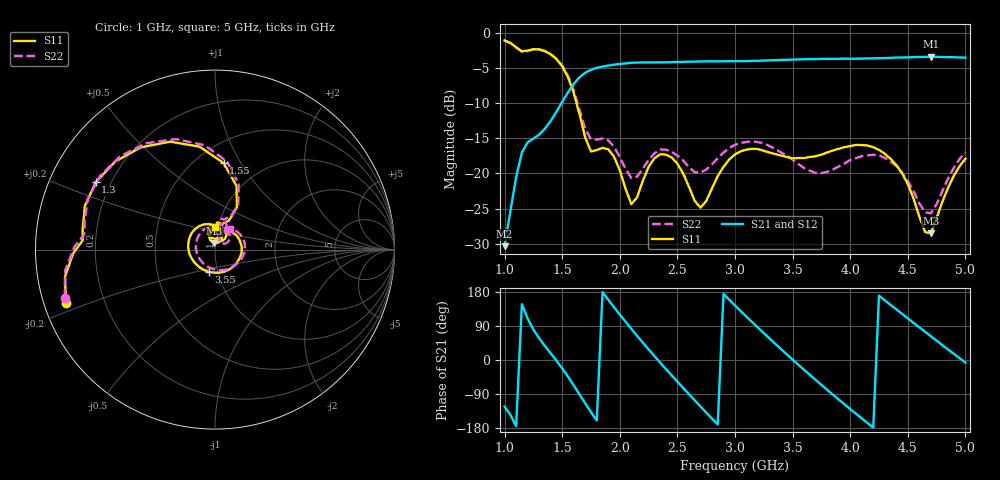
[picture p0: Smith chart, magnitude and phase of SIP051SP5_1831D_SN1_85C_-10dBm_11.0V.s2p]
# GHz  S  dB  R  50
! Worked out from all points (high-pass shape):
!   81 points, 1 GHz to 5 GHz, reference 50 ohm
!   highest |S21| = -3.41 dB at 4.7 GHz (marker M1); lowest = -30.3 dB at 1 GHz (marker M2)
!   |S21| within 3 dB of the highest: 1.645 GHz to end of sweep
!   lowest |S11| = -28.5 dB at 4.7 GHz (marker M3), VSWR 1.08, Z = 49.4 + j3.69 ohm
!   |S11| at or under -10 dB: 1.624 GHz to end of sweep
!   |S22| runs from -25.7 to -1.1 dB; largest |S21 - S12| = 0.0021
!   S11 on the Smith chart (normalised r, x): 1 GHz: 0.06, -0.17; 1.3 GHz: 0.14, +0.26; 1.55 GHz: 0.67, +0.85; 3.55 GHz: 0.91, -0.23; 5 GHz: 0.96, +0.25
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1  -1.08 -160.3  -30.34 -123.1  -30.30 -123.0  -1.10 -162.0
1.15  -2.62 176.1  -17.02 147.1  -16.99 147.3  -2.69 173.4
1.3  -2.35 150.6  -14.48 57.4  -14.47 57.3  -2.37 147.4
1.55  -6.30 84.3  -8.47 -43.9  -8.47 -43.9  -6.12 82.1
1.7  -14.91 64.2  -5.66 -114.5  -5.66 -114.6  -13.66 64.6
1.85  -16.35 85.1  -4.80 179.2  -4.79 179.3  -15.04 77.1
2.05  -22.18 68.4  -4.35 100.9  -4.34 101.0  -19.34 63.9
2.2  -21.04 112.2  -4.21 45.7  -4.21 45.7  -19.32 89.0
2.35  -17.28 90.2  -4.20 -6.6  -4.18 -6.5  -16.60 76.3
2.5  -18.61 58.6  -4.16 -57.1  -4.13 -57.1  -17.47 55.2
2.65  -23.89 50.8  -4.09 -106.3  -4.07 -106.3  -19.81 52.6
2.85  -20.38 75.8  -4.06 -170.1  -4.04 -170.1  -17.82 57.6
3  -17.28 45.1  -4.04 144.0  -4.03 144.0  -15.92 38.3
3.25  -16.78 -21.9  -3.95 70.8  -3.94 70.8  -15.71 -7.4
3.55  -17.80 -104.8  -3.77 -12.5  -3.77 -12.5  -18.66 -78.4
3.7  -17.55 -140.9  -3.73 -52.5  -3.72 -52.5  -19.92 -129.0
3.95  -16.26 165.3  -3.67 -116.8  -3.67 -116.9  -18.59 145.5
4.15  -16.02 123.8  -3.64 -166.2  -3.63 -166.3  -17.42 93.0
4.35  -17.92 84.6  -3.56 145.6  -3.56 145.7  -18.30 52.4
4.55  -23.57 58.6  -3.46 98.1  -3.45 98.1  -22.51 29.7
4.7  -28.50 96.7  -3.41 62.7  -3.41 62.7  -25.66 56.1
5  -17.92 91.2  -3.52 -6.6  -3.52 -6.7  -16.98 54.6
